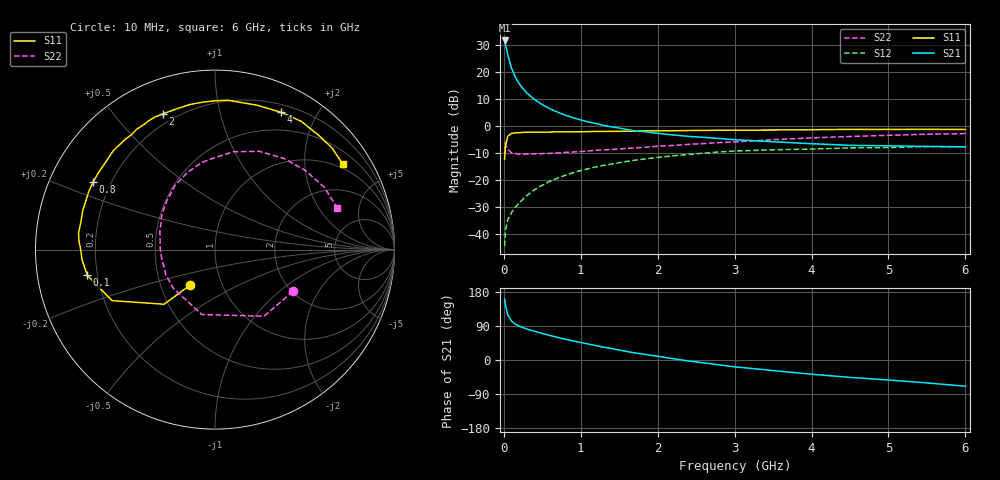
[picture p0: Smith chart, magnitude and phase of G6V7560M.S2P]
! SIEMENS Small Signal Semiconductors
! BFG193
! Si NPN RF Bipolar Junction Transistor in SOT223
! VCE = 0.75 V  IC = 60 mA
! Common Emitter S-Parameters:  August  1996
# GHz  S  MA  R  50
!  f  S11  S21  S12  S22
! GHz  MAG  ANG  MAG  ANG  MAG  ANG  MAG  ANG
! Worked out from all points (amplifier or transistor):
!   36 points, 10 MHz to 6 GHz, reference 50 ohm
!   highest |S21| = 31.5 dB at 10 MHz (marker M1)
!   |S21| within 3 dB of that: start of sweep to 33.48 MHz
!   unconditionally stable (mu >= 1): start of sweep to 18.04 MHz; 128.7 MHz to end of sweep
!   at 250 MHz: K = 1.17, MAG = 17.8 dB, |S12| = -27.0 dB
!   at 1.4 GHz: K = 1.23, MAG = 4.0 dB, |S12| = -14.1 dB
!   at 6 GHz: K = 1.08, MAG = -1.7 dB, |S12| = -7.7 dB
!   S11 on the Smith chart (normalised r, x): 10 MHz: 0.70, -0.30; 100 MHz: 0.16, -0.10; 800 MHz: 0.13, +0.25; 2 GHz: 0.15, +0.68; 4 GHz: 0.28, +1.55; 6 GHz: 0.86, +3.07
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0.01  0.2433 -125.1  37.77 161.4  0.006 70.7  0.4929 -28.2
0.02  0.4161 -133.0  33.03 146.3  0.0112 61.7  0.461 -53.7
0.05  0.6396 -153.6  20.64 119.4  0.0183 50.3  0.3688 -101.6
0.1  0.7257 -168.6  11.61 102.9  0.025 51.9  0.3166 -136.7
0.15  0.7429 -175.6  7.903 94.4  0.0313 55.7  0.3085 -152.6
0.2  0.7484 179.9  6.011 89.3  0.0379 59.5  0.2994 -161.2
0.25  0.7585 176.6  4.825 85.2  0.0447 60.7  0.3014 -168.4
0.3  0.7658 173.3  4.045 81.8  0.0518 62.6  0.3013 -172.3
0.4  0.7631 168.2  3.054 75.7  0.0661 62.8  0.3049 179.9
0.5  0.7685 163.4  2.465 70.0  0.0802 62.2  0.307 174.1
0.6  0.7689 159.1  2.067 64.7  0.0948 60.8  0.3108 169.7
0.8  0.776 151.1  1.569 54.9  0.1226 57.0  0.3243 161.2
1.1  0.7822 139.8  1.181 42.0  0.1621 50.6  0.3446 150.6
1.6  0.7998 122.9  0.852 22.5  0.2211 37.7  0.3837 134.2
2  0.8101 110.9  0.727 9.8  0.2611 27.3  0.4206 122.2
2.2  0.8129 105.3  0.68 3.5  0.2802 22.1  0.4347 116.1
2.8  0.8297 89.5  0.585 -12.8  0.3303 6.7  0.4905 98.7
3.5  0.8382 73.5  0.509 -27.9  0.361 -11.6  0.5546 79.3
4  0.8489 64.3  0.468 -37.5  0.3729 -21.1  0.6008 65.7
4.5  0.8612 56.0  0.437 -45.9  0.3917 -30.8  0.6367 52.9
5.5  0.8637 41.0  0.417 -60.4  0.4152 -52.4  0.7003 29.9
6  0.8566 33.8  0.409 -69.3  0.4105 -64.6  0.7201 18.9
